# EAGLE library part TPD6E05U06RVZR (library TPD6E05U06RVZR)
6-Channel Ultra-Low-Capacitance IEC ESD Protection Diodes Source: Datasheet
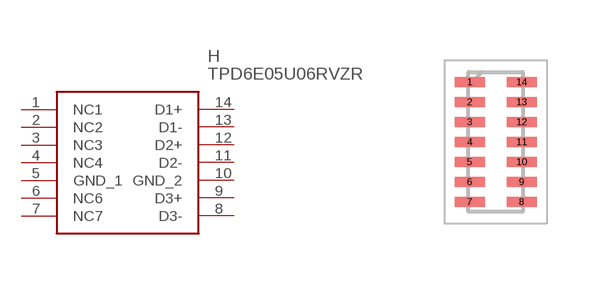
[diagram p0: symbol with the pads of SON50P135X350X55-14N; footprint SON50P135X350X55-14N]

Designator prefix H

## TPD6E05U06RVZR (Arrow_Part_Number: TPD6E05U06RVZR; Arrow_Price-Stock: https://www.arrow.com/en/products/tpd6e05u06rvzr/texas-instruments?region=nac; Description: 6-Channel Ultra-Low-Capacitance IEC ESD Protection Diodes; Height: 0.55mm; Manufacturer_Name: Texas Instruments; Manufacturer_Part_Number: TPD6E05U06RVZR; Mouser_Part_Number: 595-TPD6E05U06RVZR; Mouser_Price-Stock: https://www.mouser.co.uk/ProductDetail/Texas-Instruments/TPD6E05U06RVZR?qs=QCUnHQQYO1pCeVGx6Ibw%252BQ%3D%3D)  [SON50P135X350X55-14N]
1  NC1
2  NC2
3  NC3
4  NC4
5  GND_1  pwr
6  NC6
7  NC7
8  D3-
9  D3+
10  GND_2  pwr
11  D2-
12  D2+
13  D1-
14  D1+

## Footprint SON50P135X350X55-14N (pad centres in mm)
R-PUSON-N14
smd 0.75 x 0.25: 1 -0.65,1.5; 2 -0.65,1; 3 -0.65,0.5; 4 -0.65,0; 5 -0.65,-0.5; 6 -0.65,-1; 7 -0.65,-1.5; 8 0.65,-1.5; 9 0.65,-1; 10 0.65,-0.5; 11 0.65,0; 12 0.65,0.5; 13 0.65,1; 14 0.65,1.5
